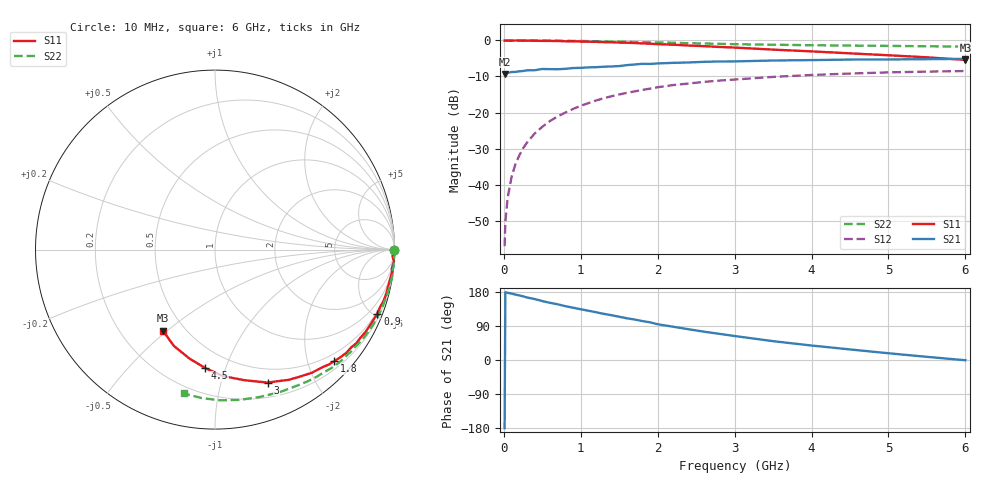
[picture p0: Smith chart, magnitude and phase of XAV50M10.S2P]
! SIEMENS Discrete & RF Semiconductors
! BFY180
! Si NPN RF Bipolar Junction Transistor in MICRO-X
! VCE = 0.5 V  IC = 0.1 mA
! Common Emitter S-Parameters:  May  1997
# GHz  S  MA  R  50
!  f  S11  S21  S12  S22
! GHz  MAG  ANG  MAG  ANG  MAG  ANG  MAG  ANG
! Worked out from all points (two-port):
!   36 points, 10 MHz to 6 GHz, reference 50 ohm
!   highest |S21| = -5.11 dB at 6 GHz (marker M1); lowest = -9.3 dB at 10 MHz (marker M2)
!   |S21| within 3 dB of the highest: 443.7 MHz to end of sweep
!   lowest |S11| = -5.4 dB at 6 GHz (marker M3), VSWR 3.32, Z = 19 - j24.2 ohm
!   |S11| at or under -10 dB: nowhere
!   |S22| runs from -1.7 to 0.0 dB; largest |S21 - S12| = 0.39
!   S11 on the Smith chart (normalised r, x): 10 MHz: open; 900 MHz: 0.40, -5.24; 1.8 GHz: 0.34, -2.49; 3 GHz: 0.35, -1.41; 4.5 GHz: 0.36, -0.85; 6 GHz: 0.38, -0.48
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0.01  0.9946 -0.2  0.342 -179.8  0.0014 82.1  0.9998 -0.1
0.02  0.9932 -0.2  0.35 178.7  0.0031 91.8  0.9999 -0.5
0.05  0.9934 -0.9  0.354 177.3  0.0066 88.1  0.9998 -1.1
0.1  0.9898 -2.2  0.365 175.2  0.0127 89.0  0.9999 -2.1
0.15  0.9994 -3.7  0.366 172.6  0.0191 86.9  0.9999 -3.2
0.2  0.9949 -4.7  0.373 170.5  0.0253 85.7  0.9981 -4.2
0.3  0.9945 -7.0  0.385 165.0  0.0382 83.4  0.9971 -6.3
0.4  0.989 -9.9  0.386 160.9  0.0511 81.3  0.9986 -8.4
0.5  0.9858 -12.0  0.402 155.5  0.0635 79.0  0.996 -10.5
0.7  0.9825 -16.9  0.399 147.0  0.0884 74.1  0.992 -14.8
0.9  0.9727 -21.5  0.414 138.0  0.1122 69.4  0.9858 -18.9
1.1  0.9608 -26.2  0.423 130.0  0.1351 65.0  0.9783 -23.1
1.4  0.9448 -33.5  0.436 118.2  0.1682 58.0  0.9665 -29.3
1.8  0.91 -43.1  0.474 102.8  0.2059 49.8  0.9459 -37.1
2.2  0.8731 -51.8  0.489 87.8  0.2404 41.5  0.9295 -44.6
2.6  0.8337 -60.5  0.505 74.8  0.2659 34.1  0.907 -51.4
3  0.7968 -68.4  0.512 63.3  0.2871 26.9  0.8878 -58.0
3.5  0.7461 -77.3  0.527 49.7  0.3121 19.7  0.8727 -65.4
4  0.7054 -86.5  0.534 38.2  0.3319 12.0  0.8584 -72.9
4.5  0.6625 -94.7  0.543 27.9  0.3475 4.9  0.8486 -80.3
5.5  0.5836 -113.1  0.55 8.3  0.3695 -8.7  0.8307 -95.1
6  0.5373 -122.7  0.555 -0.6  0.3766 -15.6  0.8203 -102.3
